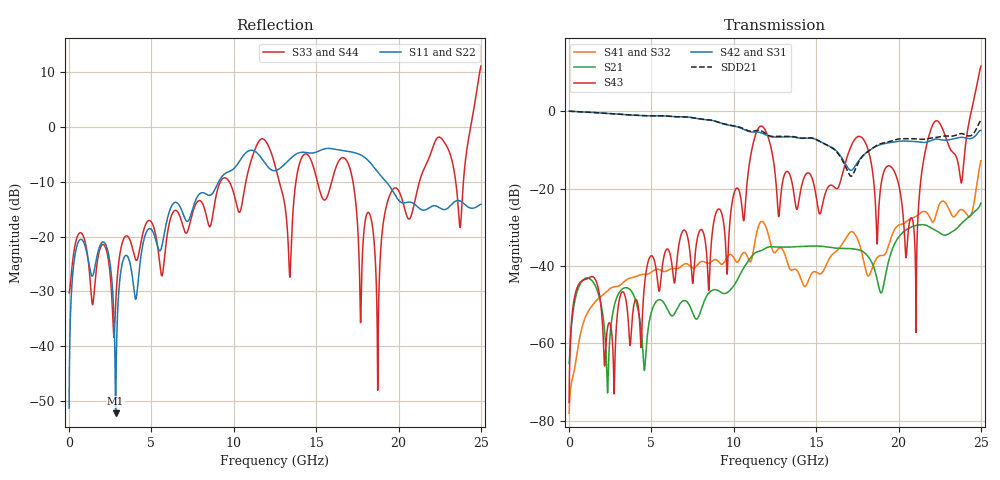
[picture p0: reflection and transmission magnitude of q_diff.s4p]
!Keysight Technologies,N5245B,MY57181346,A.12.70.07
!Automatic Fixture Removal (AFR)
!Date: Wednesday, November 07, 2018 11:52:05 AM
!S4P File: Measurements: <S11,S12,S13,S14>,
!<S21,S22,S23,S24>,
!<S31,S32,S33,S34>,
!<S41,S42,S43,S44>:
# MHz S  RI  R 50
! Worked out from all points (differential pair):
!   2499 points, 10 MHz to 24.99 GHz, reference 50 ohm
!   strongest paths, dB at 10 MHz, 6.25 GHz, 12.5 GHz, 18.75 GHz, 24.99 GHz:
!     S42: 0.0, -1.4, -6.7, -8.9, -5.0
!     S31: 0.0, -1.4, -6.7, -8.9, -5.0
!     S43: -75.3, -39.7, -15.9, -29.4, 11.6
!     S21: -65.2, -52.9, -35.1, -44.5, -23.8
!     S41: -78.1, -40.7, -36.6, -37.6, -12.8
!     S32: -78.1, -40.7, -36.6, -37.6, -12.8
!   taken as a pair (ports 2,1 in; 4,3 out), SDD21 dB: 0.0, -1.4, -6.5, -8.7, -2.5
!   lowest |S11| = -52.3 dB at 2.83 GHz (marker M1), VSWR 1.00, Z = 50 - j0.24 ohm
!   |S11| at or under -10 dB: start of sweep to 9.081 GHz; 19.25 GHz to end of sweep
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10  0.00176 0.00205  0.000543 9.01e-05  0.9996 -0.0202  0.000125 4.46e-06
    0.000543 9.01e-05  0.00176 0.00205  0.000125 4.46e-06  0.9996 -0.0202
    0.9996 -0.0202  0.000125 4.46e-06  0.0306 0.00174  -0.000114 0.000129
    0.000125 4.46e-06  0.9996 -0.0202  -0.000114 0.000129  0.0306 0.00174
1530  -0.0484 0.00595  -0.00437 -0.00397  -0.9586 -0.0649  -0.000167 -0.00331
      -0.00437 -0.00397  -0.0484 0.00595  -0.000167 -0.00331  -0.9586 -0.0649
      -0.9586 -0.0649  -0.000167 -0.00331  0.0298 0.00869  0.00552 -0.00439
      -0.000167 -0.00331  -0.9586 -0.0649  0.00552 -0.00439  0.0298 0.00869
2830  -0.000354 -0.0024  -0.00285 -0.00211  0.7528 0.5329  -0.00312 0.00443
      -0.00285 -0.00211  -0.000354 -0.0024  -0.00312 0.00443  0.7528 0.5329
      0.7528 0.5329  -0.00312 0.00443  -0.0108 0.0214  -0.000345 0.00103
      -0.00312 0.00443  0.7528 0.5329  -0.000345 0.00103  -0.0108 0.0214
11590  -0.5063 0.1924  0.0155 -0.00216  -0.1823 0.5  -0.00173 -0.036
       0.0155 -0.00216  -0.5063 0.1924  -0.00173 -0.036  -0.1823 0.5
       -0.1823 0.5  -0.00173 -0.036  -0.7564 0.1054  0.6332 -0.0443
       -0.00173 -0.036  -0.1823 0.5  0.6332 -0.0443  -0.7564 0.1054
24360  -0.0535 -0.174  0.0321 -0.0318  -0.2602 0.3586  0.00323 -0.0439
       0.0321 -0.0318  -0.0535 -0.174  0.00323 -0.0439  -0.2602 0.3586
       -0.2602 0.3586  0.00323 -0.0439  0.88 -0.4471  -0.5919 0.669
       0.00323 -0.0439  -0.2602 0.3586  -0.5919 0.669  0.88 -0.4471
24740  -0.0655 -0.1748  0.0206 -0.0493  0.0561 0.5009  -0.0556 -0.0964
       0.0206 -0.0493  -0.0655 -0.1748  -0.0556 -0.0964  0.0561 0.5009
       0.0561 0.5009  -0.0556 -0.0964  -0.8754 -1.962  1.41 1.632
       -0.0556 -0.0964  0.0561 0.5009  1.41 1.632  -0.8754 -1.962
24990  -0.099 -0.1702  0.0145 -0.0631  0.4094 0.3878  -0.2282 -0.00807
       0.0145 -0.0631  -0.099 -0.1702  -0.2282 -0.00807  0.4094 0.3878
       0.4094 0.3878  -0.2282 -0.00807  -3.539 0.6662  3.573 -1.343
       -0.2282 -0.00807  0.4094 0.3878  3.573 -1.343  -3.539 0.6662
